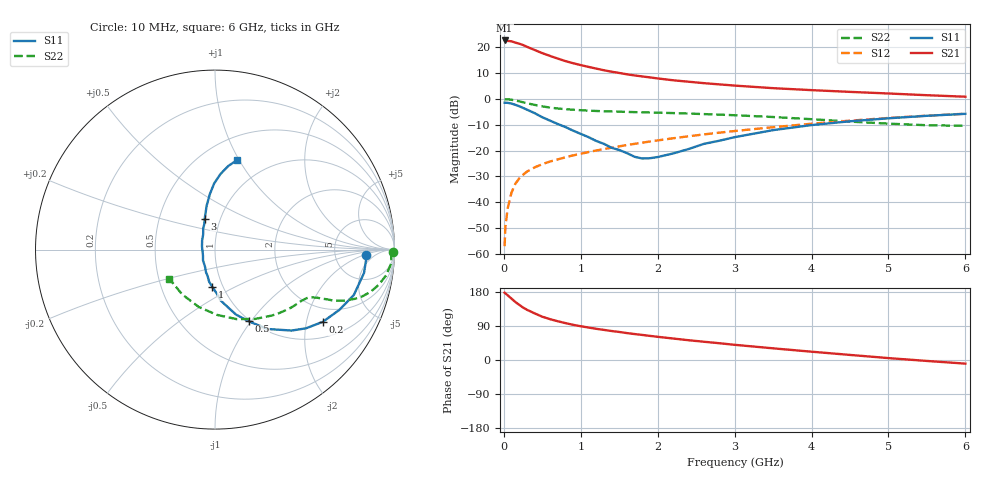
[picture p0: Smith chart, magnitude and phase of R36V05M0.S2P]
! SIEMENS Small Signal Semiconductors
! BFR181
! Si NPN RF Bipolar Junction Transistor in SOT23
! VCE = 6 V  IC = 5 mA
! Common Emitter S-Parameters:  May  1996
# GHz  S  MA  R  50
!  f  S11  S21  S12  S22
! GHz  MAG  ANG  MAG  ANG  MAG  ANG  MAG  ANG
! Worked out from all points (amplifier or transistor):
!   36 points, 10 MHz to 6 GHz, reference 50 ohm
!   highest |S21| = 22.7 dB at 10 MHz (marker M1)
!   |S21| within 3 dB of that: start of sweep to 344.2 MHz
!   unconditionally stable (mu >= 1): 1.175 GHz to 3.036 GHz
!   at 250 MHz: K = 0.41, MSG = 25.1 dB, |S12| = -29.4 dB
!   at 1.4 GHz: K = 1.04, MAG = 13.5 dB, |S12| = -18.9 dB
!   at 6 GHz: K = 0.86, MSG = 3.3 dB, |S12| = -5.7 dB
!   lowest NFmin = 1.55 dB at 450 MHz
!   S11 on the Smith chart (normalised r, x): 10 MHz: 11, -2; 200 MHz: 1.49, -2.51; 500 MHz: 0.98, -0.98; 1 GHz: 0.89, -0.39; 3 GHz: 0.84, +0.30; 6 GHz: 0.72, +0.98
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0.01  0.8438 -2.0  13.61 177.7  0.0014 90.6  0.9916 -0.8
0.02  0.8442 -3.5  13.32 175.8  0.0033 86.4  0.9817 -1.7
0.05  0.8404 -8.9  13.33 170.7  0.0076 85.0  0.9854 -4.3
0.1  0.8139 -18.1  13.1 161.9  0.0154 79.4  0.9648 -8.5
0.15  0.7697 -25.9  12.36 153.0  0.0227 75.9  0.9332 -12.1
0.2  0.7232 -33.8  11.79 145.6  0.0288 72.5  0.8996 -15.1
0.25  0.67 -40.9  11.09 138.4  0.0339 69.7  0.8613 -17.6
0.3  0.6208 -46.6  10.26 132.6  0.039 68.5  0.8261 -19.4
0.4  0.5311 -56.4  8.903 123.1  0.0471 65.5  0.7676 -21.8
0.5  0.4419 -64.8  7.724 114.2  0.0544 63.9  0.7186 -23.3
0.6  0.3803 -72.1  6.827 107.8  0.0612 63.7  0.6796 -24.0
0.7  0.3274 -77.6  6.069 102.3  0.0673 63.4  0.6538 -24.7
0.8  0.2853 -83.6  5.425 97.4  0.0739 63.3  0.6334 -25.1
1  0.2101 -93.9  4.529 89.1  0.0864 63.6  0.6048 -26.1
1.1  0.1822 -100.3  4.185 85.7  0.0935 64.1  0.5937 -26.7
1.6  0.0892 -138.6  3.005 71.0  0.1279 64.0  0.5606 -30.5
2.2  0.0878 144.9  2.302 56.7  0.173 62.4  0.5323 -37.5
3  0.1816 108.4  1.816 40.1  0.2389 57.7  0.4834 -49.6
3.5  0.2487 100.8  1.619 30.8  0.2833 53.8  0.4465 -59.9
4.5  0.3691 90.7  1.371 13.4  0.3794 43.7  0.3639 -88.2
5.5  0.4715 81.0  1.182 -2.5  0.4741 31.4  0.3095 -126.2
6  0.5149 76.0  1.105 -9.6  0.5174 24.6  0.3016 -147.4
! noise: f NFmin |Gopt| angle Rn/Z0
0.45  1.55  0.48  17  0.36
0.9  1.65  0.4  35  0.34
1.8  2  0.18  88  0.34
